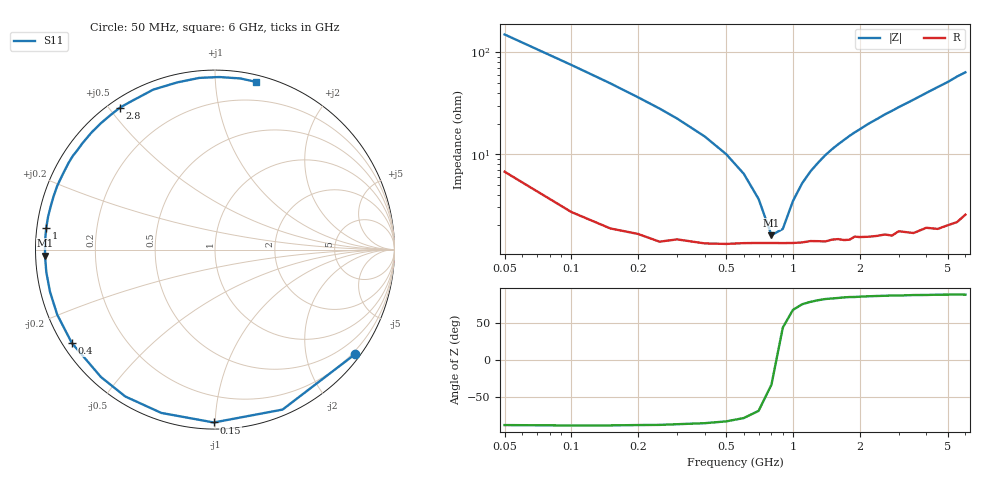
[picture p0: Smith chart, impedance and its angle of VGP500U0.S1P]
! Infineon Technologies  Discrete & RF Semiconductors
! BB 831
! Si Tuning Diode in SOD323
! VR = 0.5 V
! S-Parameters:  July  1999
# GHz  S  MA  R  50
!  f  S11
! GHz  MAG  ANG
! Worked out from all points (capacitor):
!   34 points, 50 MHz to 6 GHz, reference 50 ohm
!   read as one part to ground: C = 20.8 pF near 50 MHz
!   lowest |Z| = 1.6 ohm at 800 MHz (marker M1)
!   series resonance near 840.8 MHz, so ESL is about 1.7 nH
!   S11 on the Smith chart (normalised r, x): 50 MHz: 0.13, -3.00; 150 MHz: 0.04, -0.99; 400 MHz: 0.03, -0.30; 1 GHz: 0.03, +0.06; 2.8 GHz: 0.03, +0.53; 6 GHz: 0.05, +1.27
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0.05  0.9736 -36.8
0.1  0.9676 -67.1
0.15  0.9633 -90.4
0.2  0.9579 -108.2
0.25  0.959 -121.4
0.3  0.9528 -131.8
0.4  0.9525 -146.9
0.5  0.9509 -157.6
0.6  0.9489 -165.7
0.7  0.9481 -172.3
0.8  0.9479 -178.0
1  0.9481 172.7
1.1  0.9478 168.6
1.3  0.9472 161.5
1.4  0.948 158.1
1.6  0.9465 152.1
1.8  0.9486 146.5
1.9  0.9457 143.9
2.2  0.9482 136.5
2.4  0.9488 132.2
2.6  0.9491 127.7
2.8  0.9519 123.9
3.5  0.9554 111.1
4  0.955 102.7
4.5  0.9607 95.2
5  0.9617 88.6
5.5  0.964 81.6
6  0.962 76.2
